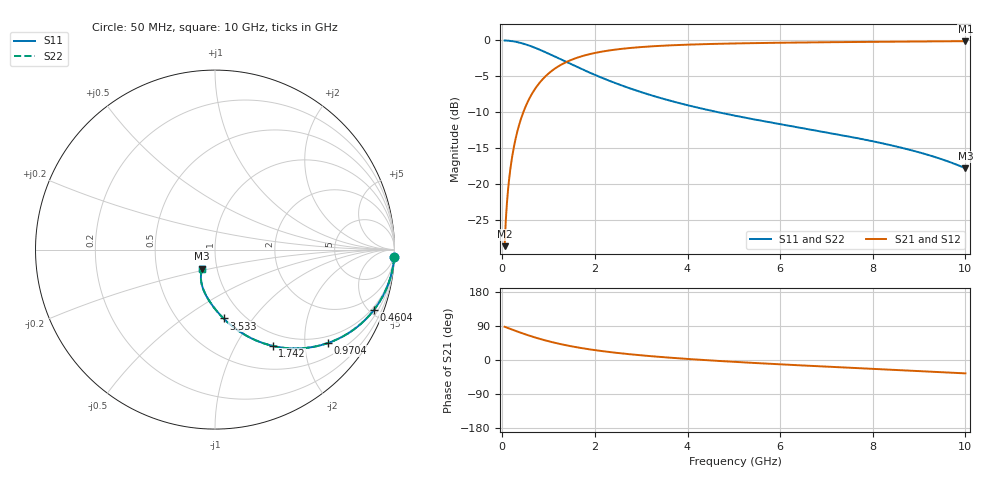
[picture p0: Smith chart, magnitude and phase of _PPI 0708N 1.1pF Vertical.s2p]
! S-Parameter data specifications (vertical orientation):
! Substrate: 40-mil Rogers 3003C, Substrate thickness, H=1.016mm, Dielectric constant, Er=3, Conductor thickness, T_mtl=0.043mm, Loss Tangent, Tand=0.003
! PCB Mounting Pad Footprint: Pad width, PadW=2.54mm , Pad length, PadL=0.51mm , Pad gap, PadG (edge-to-edge)=0.71mm , Reference planes=1.73mm apart
! Created Tue Jan 16 08:42:26 2018
# GHz S MA R 50
! 2 Port Network Data from SP1.SP block
! freq  magS11  angS11  magS21  angS21  magS12  angS12  magS22  angS22
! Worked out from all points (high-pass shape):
!   801 points, 50 MHz to 10 GHz, reference 50 ohm
!   highest |S21| = -0.11 dB at 10 GHz (marker M1); lowest = -28.7 dB at 50 MHz (marker M2)
!   |S21| within 3 dB of the highest: 1.355 GHz to end of sweep
!   lowest |S11| = -17.8 dB at 10 GHz (marker M3), VSWR 1.29, Z = 42.4 - j9.2 ohm
!   |S11| at or under -10 dB: 4.645 GHz to end of sweep
!   |S22| runs from -17.8 to 0.0 dB; largest |S21 - S12| = 0
!   S11 on the Smith chart (normalised r, x): 50 MHz: 1, -49; 460.4 MHz: 0.82, -5.35; 970.4 MHz: 0.82, -2.55; 1.742 GHz: 0.81, -1.43; 3.533 GHz: 0.81, -0.73; 10 GHz: 0.85, -0.18
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0.05  0.9993 -2.3  0.03663 87.7  0.03663 87.7  0.9993 -2.3
0.074875  0.9985 -3.5  0.05481 86.5  0.05481 86.5  0.9985 -3.5
0.1370625  0.995 -6.4  0.09997 83.6  0.09997 83.6  0.995 -6.4
0.174375  0.9919 -8.1  0.1268 81.9  0.1268 81.9  0.9919 -8.1
0.2116875  0.9882 -9.8  0.1533 80.2  0.1533 80.2  0.9882 -9.8
0.2614375  0.9821 -12.0  0.1881 78.0  0.1881 78.0  0.9821 -12.0
0.323625  0.973 -14.8  0.2307 75.2  0.2307 75.2  0.973 -14.8
0.4604375  0.9476 -20.7  0.3193 69.3  0.3193 69.3  0.9476 -20.7
0.6843125  0.8943 -29.6  0.447 60.3  0.447 60.3  0.8943 -29.6
0.970375  0.8166 -39.6  0.5767 50.4  0.5767 50.4  0.8166 -39.6
1.29375  0.7297 -48.9  0.6831 41.0  0.6831 41.0  0.7297 -48.9
1.716625  0.6303 -58.6  0.7755 31.3  0.7755 31.3  0.6303 -58.6
1.7415  0.625 -59.1  0.7797 30.8  0.7797 30.8  0.625 -59.1
2.077313  0.5609 -65.2  0.8269 24.8  0.8269 24.8  0.5609 -65.2
2.450438  0.5024 -70.8  0.8635 19.1  0.8635 19.1  0.5024 -70.8
3.370812  0.4002 -81.4  0.915 8.5  0.915 8.5  0.4002 -81.4
3.5325  0.3868 -82.9  0.9207 6.9  0.9207 6.9  0.3868 -82.9
5.025  0.2983 -94.7  0.9526 -5.0  0.9526 -5.0  0.2983 -94.7
6.691625  0.2376 -105.2  0.969 -15.7  0.969 -15.7  0.2376 -105.2
8.345812  0.187 -114.6  0.9794 -25.4  0.9794 -25.4  0.187 -114.6
9.228875  0.1576 -119.5  0.9841 -30.6  0.9841 -30.6  0.1576 -119.5
10  0.1282 -123.7  0.9878 -35.3  0.9878 -35.3  0.1282 -123.7
